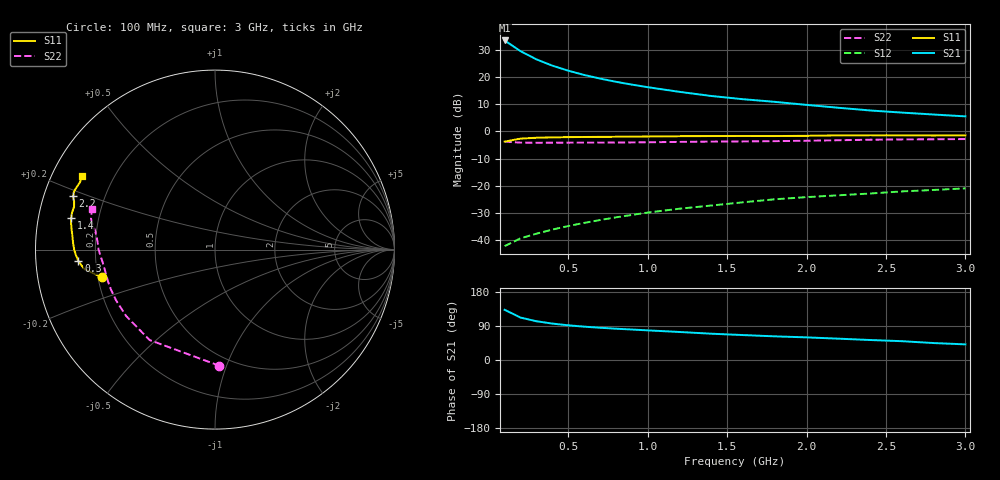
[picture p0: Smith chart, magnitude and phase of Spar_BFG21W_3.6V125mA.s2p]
! Filename: 3_6125bfg21.001
! Title: BFG21W
! Bias: Vce=3.6V; Ic=125mA
! Company: NXP Semiconductors NL
! User: Quality&Reliability T&D
! Measure time: 10 Nov 1999 / 11:44:37
#  MHz  S  MA  R 50
! Freq  S11  S21  S12  S22  :
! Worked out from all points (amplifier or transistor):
!   20 points, 100 MHz to 3 GHz, reference 50 ohm
!   highest |S21| = 33.4 dB at 100 MHz (marker M1)
!   |S21| within 3 dB of that: start of sweep to 176.5 MHz
!   unconditionally stable (mu >= 1): 632.7 MHz to end of sweep
!   at 400 MHz: K = 0.90, MSG = 30.1 dB, |S12| = -36.1 dB
!   at 1.2 GHz: K = 1.06, MAG = 20.0 dB, |S12| = -28.4 dB
!   at 3 GHz: K = 1.05, MAG = 11.9 dB, |S12| = -20.9 dB
!   S11 on the Smith chart (normalised r, x): 100 MHz: 0.22, -0.12; 300 MHz: 0.13, -0.04; 1.4 GHz: 0.10, +0.11; 2.2 GHz: 0.09, +0.18; 3 GHz: 0.09, +0.26
100  0.6474 -166.2  46.74 132.6  0.007798 56.2  0.6478 -87.8
200  0.7366 -171.5  29.76 112.0  0.01087 53.5  0.6219 -125.9
300  0.7639 -175.3  21.03 102.3  0.01321 56.7  0.6179 -143.2
400  0.7764 -177.9  16.13 96.1  0.01572 60.2  0.6195 -152.7
500  0.7841 -179.9  13.03 91.6  0.01825 63.2  0.6208 -158.9
600  0.789 178.3  10.88 88.0  0.02084 65.4  0.6219 -163.2
700  0.7929 176.6  9.337 85.1  0.02355 67.4  0.6224 -166.5
800  0.7965 175.1  8.15 82.6  0.02636 68.9  0.624 -169.3
900  0.8009 173.6  7.226 80.5  0.0292 70.5  0.627 -171.8
1000  0.806 172.2  6.487 78.2  0.03228 71.1  0.6309 -174.0
1200  0.815 169.8  5.322 74.0  0.038 72.1  0.6408 -177.5
1400  0.8204 167.7  4.467 69.4  0.0435 72.4  0.6494 179.7
1600  0.8227 165.5  3.899 65.8  0.04986 72.5  0.6539 177.1
1800  0.8207 163.1  3.486 62.4  0.05662 72.5  0.6616 174.4
2000  0.8289 161.2  3.066 59.7  0.06203 73.1  0.6732 171.6
2200  0.8448 159.3  2.716 56.3  0.06699 72.7  0.6878 169.3
2400  0.8498 157.6  2.421 52.8  0.07226 71.9  0.7023 167.6
2600  0.8458 155.8  2.215 49.6  0.07901 70.8  0.7117 166.1
2800  0.8408 153.4  2.04 44.7  0.08397 69.0  0.7159 164.1
3000  0.8451 150.9  1.887 41.2  0.08984 68.1  0.7227 161.6
